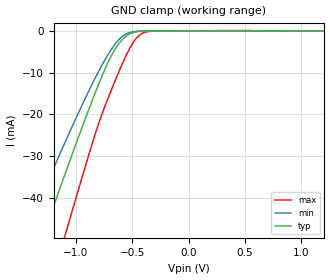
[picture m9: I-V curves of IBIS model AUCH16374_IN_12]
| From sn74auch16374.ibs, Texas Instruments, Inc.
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[Model]   AUCH16374_IN_12
Model_type  Input
Vinl=0.385
Vinh=0.845
| variable   typ   min   max
C_comp   2.81pF   2.28pF   3.21pF
[Temperature Range]   40   100   -40
| Ambient temperature   25   85   -40
[Voltage range]   1.2   1.1   1.3
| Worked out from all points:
|   GND clamp passes 1 mA (typ) near -0.54 V on its own axis
[GND Clamp]
| AUCH16374_IN_12
|   Voltage   I(typ)   I(min)   I(max)
-3.6V     -229mA     -190.7mA   -276.9mA
-1.455V   -61.51mA   -48.84mA   -81.86mA
-1.41V    -58.04mA   -45.99mA   -77.71mA
-1.28V    -48.06mA   -37.84mA   -65.72mA
-1.115V   -35.54mA   -27.71mA   -50.49mA
-1.075V   -32.55mA   -25.31mA   -46.81mA
-835mV    -15.19mA   -11.56mA   -25.12mA
-695mV    -6.412mA   -4.794mA   -14.74mA
-575mV    -1.739mA   -1.073mA   -7.038mA
-430mV    -126.3uA   -66.76uA   -901.1uA
-300mV    -34.37uA   -20.83uA   -74.27uA
1.2V      152.4pA    532.7nA    33.85pA
